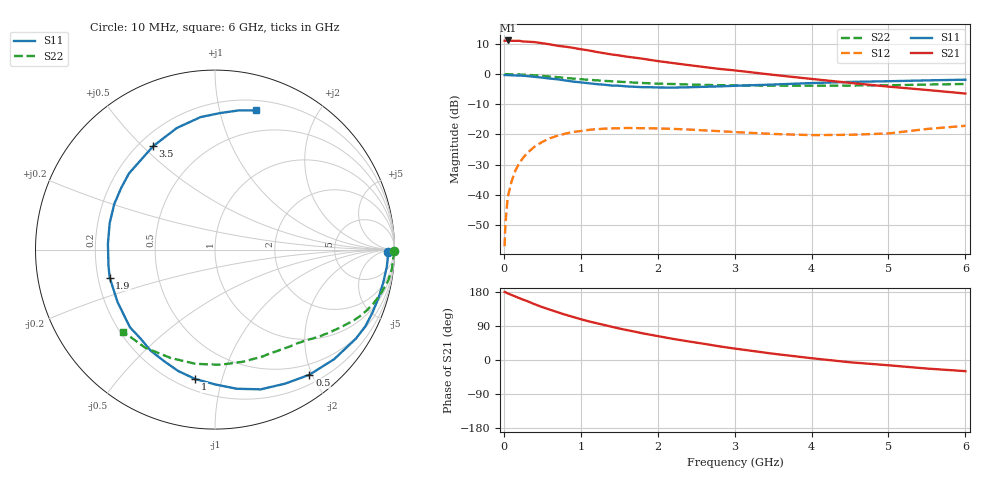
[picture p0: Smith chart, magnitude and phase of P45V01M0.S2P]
! SIEMENS Small Signal Semiconductors
! BFP182
! Si NPN RF Bipolar Junction Transistor in SOT143
! VCE = 5 V  IC = 1 mA
! Common Emitter S-Parameters:  March  1996
# GHz  S  MA  R  50
!  f  S11  S21  S12  S22
! GHz  MAG  ANG  MAG  ANG  MAG  ANG  MAG  ANG
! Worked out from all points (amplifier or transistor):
!   36 points, 10 MHz to 6 GHz, reference 50 ohm
!   highest |S21| = 11.2 dB at 50 MHz (marker M1)
!   |S21| within 3 dB of that: start of sweep to 1.024 GHz
!   unconditionally stable (mu >= 1): 2.66 GHz to end of sweep
!   at 250 MHz: K = 0.09, MSG = 19.3 dB, |S12| = -27.8 dB
!   at 1.4 GHz: K = 0.53, MSG = 12.3 dB, |S12| = -18.0 dB
!   at 6 GHz: K = 1.07, MAG = 3.7 dB, |S12| = -17.1 dB
!   S11 on the Smith chart (normalised r, x): 10 MHz: 48, -22; 500 MHz: 0.33, -1.96; 1 GHz: 0.27, -0.82; 1.9 GHz: 0.25, -0.12; 3.5 GHz: 0.26, +0.54; 6 GHz: 0.29, +1.30
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0.01  0.9658 -0.9  3.576 179.5  0.0014 92.9  0.9982 -0.4
0.02  0.9641 -2.3  3.568 179.0  0.0032 89.6  0.9967 -0.8
0.05  0.962 -5.6  3.616 175.8  0.009 90.7  0.9962 -1.9
0.1  0.9556 -10.9  3.571 171.7  0.0166 82.1  0.9919 -4.0
0.2  0.9448 -21.9  3.57 163.3  0.0332 76.7  0.9861 -8.0
0.4  0.902 -42.6  3.395 147.2  0.0627 63.7  0.9532 -15.4
0.5  0.8733 -53.0  3.255 139.5  0.0751 57.3  0.9324 -18.8
0.6  0.8432 -62.3  3.112 132.7  0.0864 52.2  0.9111 -21.8
0.8  0.7847 -81.1  2.852 119.5  0.103 41.9  0.8665 -27.2
1  0.7294 -98.7  2.587 107.7  0.1139 33.4  0.8233 -31.8
1.1  0.7067 -106.9  2.476 102.2  0.1186 30.1  0.8047 -33.7
1.3  0.6677 -122.5  2.225 92.6  0.1242 23.2  0.7735 -37.5
1.5  0.642 -137.5  2.041 83.1  0.1264 17.6  0.7469 -40.8
1.8  0.6075 -158.7  1.803 70.6  0.1268 11.2  0.7124 -45.3
1.9  0.607 -165.1  1.722 66.9  0.1265 8.9  0.7042 -47.1
2.2  0.5974 177.0  1.524 55.7  0.1235 4.2  0.6845 -51.7
2.8  0.6255 146.8  1.221 36.1  0.1132 -1.1  0.6547 -61.9
3.5  0.6715 120.9  0.973 16.6  0.1017 -1.6  0.6439 -75.9
4  0.7102 107.4  0.832 4.7  0.0973 2.7  0.6423 -87.3
4.5  0.7427 96.2  0.716 -6.0  0.0985 7.6  0.6457 -99.7
5.5  0.7868 80.3  0.546 -22.6  0.123 16.8  0.6709 -125.5
6  0.8082 73.6  0.476 -29.4  0.1389 15.7  0.686 -138.2
